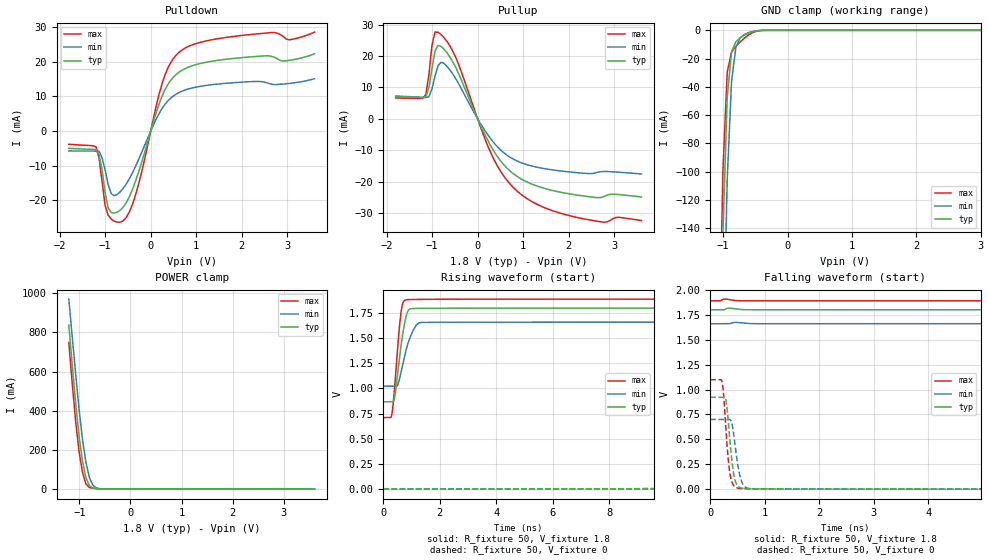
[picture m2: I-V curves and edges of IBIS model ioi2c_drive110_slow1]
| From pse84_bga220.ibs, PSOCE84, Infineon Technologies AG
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[Model] ioi2c_drive110_slow1
Model_type I/O
Enable   Active-High
Vinl  =  0.54
Vinh  =  1.26
Vmeas =  0.9
Cref  =  15e-12
| Capacitance   typ   min   max
C_comp   8.55364e-13 8.30808e-13 8.84570e-13
| Variables   typ   min   max
[GND Clamp Reference]   0   0   0
[POWER Clamp Reference]   1.8   1.66   1.89
[Pulldown Reference]   0   0   0
[Pullup Reference]   1.8   1.66   1.89
[Temperature Range]   25   125   -40
[Voltage Range]   1.8   1.66   1.89
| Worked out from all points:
|   slope of the pulldown table from 0 to 0.27 V, typ, clamps not added: 25.3 ohm
|   slope of the pullup table from 0 to 0.27 V, typ, clamps not added: 33.2 ohm
|   GND clamp passes 1 mA (typ) near -0.55 V on its own axis
|   POWER clamp passes 1 mA (typ) near -0.55 V on its own axis
|   falling waveform, R_fixture 50, V_fixture 1.8: 20-80 % time 94.6ns typ, 141ns min, 54.9ns max; typ from 1.8 V to 0.867 V
|   falling waveform, R_fixture 50, V_fixture 0: 20-80 % time 98.7ps typ, 114ps min, 90.3ps max; typ from 0.922 V to 0 V
|   rising waveform, R_fixture 50, V_fixture 1.8: 20-80 % time 261ps typ, 367ps min, 204ps max; typ from 0.867 V to 1.8 V
|   rising waveform, R_fixture 50, V_fixture 0: 20-80 % time 100ns typ, 152ns min, 59.7ns max; typ from 0 V to 0.922 V
[GND Clamp]
| Voltage   I(typ)   I(min)   I(max)
-1.204V   -750.5mA   -844.3mA   -692.2mA
-1.07V    -311.8mA   -416.8mA   -250.3mA
-1.003V   -144.6mA   -236.7mA   -99.35mA
-936.6mV  -47.15mA   -105.3mA   -29.57mA
-869.7mV  -15.32mA   -36.11mA   -15.4mA
-802.8mV  -8.178mA   -12.13mA   -11.32mA
-735.9mV  -5.345mA   -5.294mA   -8.218mA
-669mV    -3.361mA   -2.852mA   -5.471mA
-535.2mV  -838.5uA   -772.4uA   -1.486mA
-401.4mV  -47.36uA   -84.85uA   -76.78uA
3.6V      0A         0A         0A
[POWER Clamp]
| Voltage   I(typ)   I(min)   I(max)
-1.204V   837.3mA    970.7mA    749.2mA
-1.137V   634.9mA    778.2mA    540.5mA
-1.07V    440.1mA    587.4mA    346.5mA
-1.003V   270mA      407mA      190.9mA
-936.6mV  141.8mA    252.7mA    85.92mA
-869.7mV  58.74mA    136.5mA    26.66mA
-802.8mV  18.35mA    60.36mA    8.197mA
-735.9mV  5.885mA    21mA       4.755mA
-669mV    2.866mA    6.628mA    3.138mA
-334.5mV  12.31uA    45.7uA     5.857uA
3.6V      0A         0A         0A
[Pulldown]
| Voltage   I(typ)   I(min)   I(max)
-1.8V     -5.032mA   -5.777mA   -3.871mA
-1.204V   -5.387mA   -5.827mA   -4.579mA
-1.07V    -11.23mA   -7.715mA   -14.5mA
-1.003V   -17.74mA   -11.24mA   -21.48mA
-936.6mV  -22.19mA   -15.46mA   -24.35mA
-802.8mV  -23.75mA   -18.74mA   -26.09mA
-669mV    -22.91mA   -17.59mA   -26.38mA
-401.4mV  -16.91mA   -12.1mA    -21.21mA
248.3mV   10.03mA    6.478mA    13.65mA
558.6mV   16.35mA    10.65mA    21.94mA
1.49V     20.45mA    13.59mA    26.71mA
3.6V      22.33mA    15.11mA    28.59mA
[Pullup]
| Voltage   I(typ)   I(min)   I(max)
-1.8V     7.004mA    7.257mA    6.624mA
-1.137V   7.076mA    6.755mA    7.789mA
-1.07V    9.87mA     7.025mA    14.05mA
-1.003V   15.97mA    9.494mA    23.33mA
-936.6mV  21.5mA     13.55mA    27.61mA
-869.7mV  23.39mA    16.92mA    27.57mA
-735.9mV  22.13mA    17.61mA    25.79mA
-468.3mV  15.97mA    12.49mA    19.13mA
372.4mV   -10.69mA   -7.889mA   -13.34mA
869mV     -18.35mA   -13.44mA   -23.02mA
2.126V    -24.16mA   -17.07mA   -31.22mA
3.6V      -24.91mA   -17.57mA   -32.41mA
[Ramp]
dV/dt_r   0.553132/0.10019u  0.419462/0.151552u  0.659215/59.7042n
dV/dt_f   0.559853/94.5679n  0.382199/0.141345u  0.708159/54.9103n
R_load = 50
[Falling Waveform]
R_fixture = 50
V_fixture = 1.8
V_fixture_min = 1.66
V_fixture_max = 1.89
| Time   V(typ)   V(min)   V(max)
0s        1.8V       1.66V      1.89V
10.17ns   1.8V       1.66V      1.861V
20.88ns   1.758V     1.657V     1.647V
39.63ns   1.584V     1.607V     1.31V
62.21ns   1.392V     1.513V     1.044V
87.29ns   1.229V     1.412V     880.4mV
129.1ns   1.059V     1.281V     766.1mV
199.5ns   933.2mV    1.15V      719.2mV
320.7ns   877.9mV    1.06V      710.2mV
800ns     866.9mV    1.023V     709.7mV
[Falling Waveform]
R_fixture = 50
V_fixture = 0
V_fixture_min = 0
V_fixture_max = 0
| Time   V(typ)   V(min)   V(max)
0s        921.9mV    699.8mV    1.099V
216.4ps   921.7mV    699.8mV    1.076V
244.4ps   922.1mV    699.8mV    947.8mV
286.5ps   890.6mV    699.7mV    604.9mV
341.5ps   605mV      700.2mV    232.4mV
434.3ps   137.5mV    531.1mV    32.43mV
533.9ps   19.03mV    157.6mV    8.124mV
640.6ps   5.43mV     22.04mV    5.238mV
1.655ns   1.586mV    1.32mV     1.568mV
800ns     6.846nV    468.5nV    2.545nV
[Rising Waveform]
R_fixture = 50
V_fixture = 1.8
V_fixture_min = 1.66
V_fixture_max = 1.89
| Time   V(typ)   V(min)   V(max)
0s        866.9mV    1.023V     709.7mV
302.4ps   867mV      1.023V     746.8mV
412.6ps   938mV      1.023V     1.062V
566.5ps   1.294V     1.09V      1.607V
632ps     1.441V     1.171V     1.773V
691ps     1.552V     1.248V     1.853V
878.6ps   1.776V     1.455V     1.885V
1.157ns   1.797V     1.627V     1.886V
1.946ns   1.798V     1.659V     1.888V
800ns     1.8V       1.66V      1.89V
[Rising Waveform]
R_fixture = 50
V_fixture = 0
V_fixture_min = 0
V_fixture_max = 0
| Time   V(typ)   V(min)   V(max)
0s        6.812nV    466.6nV    2.54nV
12ns      51.67uV    -114.3uV   21.06mV
22.77ns   38.35mV    4.928mV    192.4mV
41.56ns   195.2mV    58.06mV    492.8mV
68.52ns   408.6mV    173.8mV    779.3mV
93.6ns    560.2mV    275.2mV    924.3mV
135.4ns   723.3mV    409.8mV    1.032V
212.8ns   855mV      560mV      1.086V
329.8ns   907.9mV    652.9mV    1.097V
800ns     921.9mV    699.1mV    1.099V
